FUNCTION "CAMS_PRESS" : VOID
TITLE =CAMS PRESS
AUTHOR : Esposito
FAMILY : EGAL_srl
NAME : CAMS_P
VERSION : 0.1


VAR_TEMP
  Cam_0_ON : BOOL ;
  Cam_0_OFF : BOOL ;
  Cam_1_on : BOOL ;
  Cam_1_OFF : BOOL ;
  Cam_2_ON : BOOL ;
  Cam_2_OFF : BOOL ;
  Cam_3_ON : BOOL ;
  Cam_3_OFF : BOOL ;
  Cam_4_ON : BOOL ;
  Cam_4_OFF : BOOL ;
  Cam_5_ON : BOOL ;
  Cam_5_OFF : BOOL ;
  Cam_6_ON : BOOL ;
  Cam_6_OFF : BOOL ;
  Cam_7_ON : BOOL ;
  Cam_7_OFF : BOOL ;
  Cam_8_ON : BOOL ;
  Cam_8_OFF : BOOL ;
  Cam_9_ON : BOOL ;
  Cam_9_OFF : BOOL ;
  Cam_10_ON : BOOL ;
  Cam_10_OFF : BOOL ;
  Cam_11_ON : BOOL ;
  Cam_11_OFF : BOOL ;
  Cam_12_ON : BOOL ;
  Cam_12_OFF : BOOL ;
  LD_K_parts : DINT ;
  LD_COUNT_R1 : DINT ;
  LD_COUNT_R2 : DINT ;
END_VAR
BEGIN
NETWORK
TITLE =LOAD AND TRANSFER VALUE K_PARTS COUNTERS

      U     "M_m1.0";
      SPBNB _001;
      L     "DB_TD_OP37".K_parts_counter;
      T     #LD_K_parts;
_001: NOP   0;
NETWORK
TITLE =LOAD VALUE COUNTER FROM ROBOT 1 AND 2

      U     "M_m1.0";
      =     L     16.0;
      U     L     16.0;
      SPBNB _002;
      L     "DB_SERVICE".VALUE_ROB1;
      T     #LD_COUNT_R1;
_002: NOP   0;
      U     L     16.0;
      SPBNB _003;
      L     "DB_SERVICE".VALUE_ROB2;
      T     #LD_COUNT_R2;
_003: NOP   0;
NETWORK
TITLE =COMPARE VALUES AND LOAD FORMULATION CAM_0

      U     "M_m1.0";
      =     L     16.0;
      U     L     16.0;
      U(    ;
      L     "DB_TD_OP37".Elec_Num_prog;
      L     0;
      ==I   ;
      )     ;
      U     "M_m21.1";
      =     L     16.1;
      U     L     16.1;
      SPBNB _004;
      L     "DB_TD_OP37".Elec_Start_prog;
      T     "DB_TD_OP37".Elec_cam_ON0;
_004: NOP   0;
      U     L     16.1;
      SPBNB _005;
      L     "DB_TD_OP37".Elec_Stop_prog;
      T     "DB_TD_OP37".Elec_cam_OFF0;
_005: NOP   0;
      U     L     16.0;
      U     "M_m21.1";
      U     ==0;
      =     L     16.1;
      U     L     16.1;
      U(    ;
      L     "DB_TD_OP37".Elec_Start_prog;
      L     "DB_TD_OP37".Elec_cam_ON0;
      ==I   ;
      )     ;
      =     #Cam_0_ON;
      U     L     16.1;
      U(    ;
      L     "DB_TD_OP37".Elec_Stop_prog;
      L     "DB_TD_OP37".Elec_cam_OFF0;
      ==I   ;
      )     ;
      =     #Cam_0_OFF;
      U     L     16.0;
      U     #Cam_0_ON;
      U     #Cam_0_OFF;
      R     "M_m21.1";
NETWORK
TITLE =COMPARE VALUES AND LOAD FORMULATION CAM_1

      U     "M_m1.0";
      =     L     16.0;
      U     L     16.0;
      U(    ;
      L     "DB_TD_OP37".Elec_Num_prog;
      L     1;
      ==I   ;
      )     ;
      U     "M_m21.1";
      =     L     16.1;
      U     L     16.1;
      SPBNB _006;
      L     "DB_TD_OP37".Elec_Start_prog;
      T     "DB_TD_OP37".Elec_cam_ON1;
_006: NOP   0;
      U     L     16.1;
      SPBNB _007;
      L     "DB_TD_OP37".Elec_Stop_prog;
      T     "DB_TD_OP37".Elec_cam_OFF1;
_007: NOP   0;
      U     L     16.0;
      U     "M_m21.1";
      U     ==0;
      =     L     16.1;
      U     L     16.1;
      U(    ;
      L     "DB_TD_OP37".Elec_Start_prog;
      L     "DB_TD_OP37".Elec_cam_ON1;
      ==I   ;
      )     ;
      =     #Cam_1_on;
      U     L     16.1;
      U(    ;
      L     "DB_TD_OP37".Elec_Stop_prog;
      L     "DB_TD_OP37".Elec_cam_OFF1;
      ==I   ;
      )     ;
      =     #Cam_1_OFF;
      U     L     16.0;
      U     #Cam_1_on;
      U     #Cam_1_OFF;
      R     "M_m21.1";
NETWORK
TITLE =COMPARE VALUES AND LOAD FORMULATION CAM_2

      U     "M_m1.0";
      =     L     16.0;
      U     L     16.0;
      U(    ;
      L     "DB_TD_OP37".Elec_Num_prog;
      L     2;
      ==I   ;
      )     ;
      U     "M_m21.1";
      =     L     16.1;
      U     L     16.1;
      SPBNB _008;
      L     "DB_TD_OP37".Elec_Start_prog;
      T     "DB_TD_OP37".Elec_cam_ON2;
_008: NOP   0;
      U     L     16.1;
      SPBNB _009;
      L     "DB_TD_OP37".Elec_Stop_prog;
      T     "DB_TD_OP37".Elec_cam_OFF2;
_009: NOP   0;
      U     L     16.0;
      U     "M_m21.1";
      U     ==0;
      =     L     16.1;
      U     L     16.1;
      U(    ;
      L     "DB_TD_OP37".Elec_Start_prog;
      L     "DB_TD_OP37".Elec_cam_ON2;
      ==I   ;
      )     ;
      =     #Cam_2_ON;
      U     L     16.1;
      U(    ;
      L     "DB_TD_OP37".Elec_Stop_prog;
      L     "DB_TD_OP37".Elec_cam_OFF2;
      ==I   ;
      )     ;
      =     #Cam_2_OFF;
      U     L     16.0;
      U     #Cam_2_ON;
      U     #Cam_2_OFF;
      R     "M_m21.1";
NETWORK
TITLE =COMPARE VALUES AND LOAD FORMULATION CAM_3

      U     "M_m1.0";
      =     L     16.0;
      U     L     16.0;
      U(    ;
      L     "DB_TD_OP37".Elec_Num_prog;
      L     3;
      ==I   ;
      )     ;
      U     "M_m21.1";
      =     L     16.1;
      U     L     16.1;
      SPBNB _00a;
      L     "DB_TD_OP37".Elec_Start_prog;
      T     "DB_TD_OP37".Elec_cam_ON3;
_00a: NOP   0;
      U     L     16.1;
      SPBNB _00b;
      L     "DB_TD_OP37".Elec_Stop_prog;
      T     "DB_TD_OP37".Elec_cam_OFF3;
_00b: NOP   0;
      U     L     16.0;
      U     "M_m21.1";
      U     ==0;
      =     L     16.1;
      U     L     16.1;
      U(    ;
      L     "DB_TD_OP37".Elec_Start_prog;
      L     "DB_TD_OP37".Elec_cam_ON3;
      ==I   ;
      )     ;
      =     #Cam_3_ON;
      U     L     16.1;
      U(    ;
      L     "DB_TD_OP37".Elec_Stop_prog;
      L     "DB_TD_OP37".Elec_cam_OFF3;
      ==I   ;
      )     ;
      =     #Cam_3_OFF;
      U     L     16.0;
      U     #Cam_3_ON;
      U     #Cam_3_OFF;
      R     "M_m21.1";
NETWORK
TITLE =COMPARE VALUES AND LOAD FORMULATION CAM_4

      U     "M_m1.0";
      =     L     16.0;
      U     L     16.0;
      U(    ;
      L     "DB_TD_OP37".Elec_Num_prog;
      L     4;
      ==I   ;
      )     ;
      U     "M_m21.1";
      =     L     16.1;
      U     L     16.1;
      SPBNB _00c;
      L     "DB_TD_OP37".Elec_Start_prog;
      T     "DB_TD_OP37".Elec_cam_ON4;
_00c: NOP   0;
      U     L     16.1;
      SPBNB _00d;
      L     "DB_TD_OP37".Elec_Stop_prog;
      T     "DB_TD_OP37".Elec_cam_OFF4;
_00d: NOP   0;
      U     L     16.0;
      U     "M_m21.1";
      U     ==0;
      =     L     16.1;
      U     L     16.1;
      U(    ;
      L     "DB_TD_OP37".Elec_Start_prog;
      L     "DB_TD_OP37".Elec_cam_ON4;
      ==I   ;
      )     ;
      =     #Cam_4_ON;
      U     L     16.1;
      U(    ;
      L     "DB_TD_OP37".Elec_Stop_prog;
      L     "DB_TD_OP37".Elec_cam_OFF4;
      ==I   ;
      )     ;
      =     #Cam_4_ON;
      U     L     16.0;
      U     #Cam_4_ON;
      U     #Cam_4_OFF;
      R     "M_m21.1";
NETWORK
TITLE =COMPARE VALUES AND LOAD FORMULATION CAM_5

      U     "M_m1.0";
      =     L     16.0;
      U     L     16.0;
      U(    ;
      L     "DB_TD_OP37".Elec_Num_prog;
      L     5;
      ==I   ;
      )     ;
      U     "M_m21.1";
      =     L     16.1;
      U     L     16.1;
      SPBNB _00e;
      L     "DB_TD_OP37".Elec_Start_prog;
      T     "DB_TD_OP37".Elec_cam_ON5;
_00e: NOP   0;
      U     L     16.1;
      SPBNB _00f;
      L     "DB_TD_OP37".Elec_Stop_prog;
      T     "DB_TD_OP37".Elec_cam_OFF5;
_00f: NOP   0;
      U     L     16.0;
      U     "M_m21.1";
      U     ==0;
      =     L     16.1;
      U     L     16.1;
      U(    ;
      L     "DB_TD_OP37".Elec_Start_prog;
      L     "DB_TD_OP37".Elec_cam_ON5;
      ==I   ;
      )     ;
      =     #Cam_5_ON;
      U     L     16.1;
      U(    ;
      L     "DB_TD_OP37".Elec_Stop_prog;
      L     "DB_TD_OP37".Elec_cam_OFF5;
      ==I   ;
      )     ;
      =     #Cam_5_OFF;
      U     L     16.0;
      U     #Cam_5_ON;
      U     #Cam_5_OFF;
      R     "M_m21.1";
NETWORK
TITLE =COMPARE VALUES AND LOAD FORMULATION CAM_6

      U     "M_m1.0";
      =     L     16.0;
      U     L     16.0;
      U(    ;
      L     "DB_TD_OP37".Elec_Num_prog;
      L     6;
      ==I   ;
      )     ;
      U     "M_m21.1";
      =     L     16.1;
      U     L     16.1;
      SPBNB _010;
      L     "DB_TD_OP37".Elec_Start_prog;
      T     "DB_TD_OP37".Elec_cam_ON6;
_010: NOP   0;
      U     L     16.1;
      SPBNB _011;
      L     "DB_TD_OP37".Elec_Stop_prog;
      T     "DB_TD_OP37".Elec_cam_OFF6;
_011: NOP   0;
      U     L     16.0;
      U     "M_m21.1";
      U     ==0;
      =     L     16.1;
      U     L     16.1;
      U(    ;
      L     "DB_TD_OP37".Elec_Start_prog;
      L     "DB_TD_OP37".Elec_cam_ON6;
      ==I   ;
      )     ;
      =     #Cam_6_ON;
      U     L     16.1;
      U(    ;
      L     "DB_TD_OP37".Elec_Stop_prog;
      L     "DB_TD_OP37".Elec_cam_OFF6;
      ==I   ;
      )     ;
      =     #Cam_6_OFF;
      U     L     16.0;
      U     #Cam_6_ON;
      U     #Cam_6_OFF;
      R     "M_m21.1";
NETWORK
TITLE =COMPARE VALUES AND LOAD FORMULATION CAM_7

      U     "M_m1.0";
      =     L     16.0;
      U     L     16.0;
      U(    ;
      L     "DB_TD_OP37".Elec_Num_prog;
      L     7;
      ==I   ;
      )     ;
      U     "M_m21.1";
      =     L     16.1;
      U     L     16.1;
      SPBNB _012;
      L     "DB_TD_OP37".Elec_Start_prog;
      T     "DB_TD_OP37".Elec_cam_ON7;
_012: NOP   0;
      U     L     16.1;
      SPBNB _013;
      L     "DB_TD_OP37".Elec_Stop_prog;
      T     "DB_TD_OP37".Elec_cam_OFF7;
_013: NOP   0;
      U     L     16.0;
      U     "M_m21.1";
      U     ==0;
      =     L     16.1;
      U     L     16.1;
      U(    ;
      L     "DB_TD_OP37".Elec_Start_prog;
      L     "DB_TD_OP37".Elec_cam_ON7;
      ==I   ;
      )     ;
      =     #Cam_7_ON;
      U     L     16.1;
      U(    ;
      L     "DB_TD_OP37".Elec_cam_OFF7;
      L     "DB_TD_OP37".Elec_cam_OFF2;
      ==I   ;
      )     ;
      =     #Cam_7_OFF;
      U     L     16.0;
      U     #Cam_7_ON;
      U     #Cam_7_OFF;
      R     "M_m21.1";
NETWORK
TITLE =COMPARE VALUES AND LOAD FORMULATION CAM_8

      U     "M_m1.0";
      =     L     16.0;
      U     L     16.0;
      U(    ;
      L     "DB_TD_OP37".Elec_Num_prog;
      L     8;
      ==I   ;
      )     ;
      U     "M_m21.1";
      =     L     16.1;
      U     L     16.1;
      SPBNB _014;
      L     "DB_TD_OP37".Elec_Start_prog;
      T     "DB_TD_OP37".Elec_cam_ON8;
_014: NOP   0;
      U     L     16.1;
      SPBNB _015;
      L     "DB_TD_OP37".Elec_Stop_prog;
      T     "DB_TD_OP37".Elec_cam_OFF8;
_015: NOP   0;
      U     L     16.0;
      U     "M_m21.1";
      U     ==0;
      =     L     16.1;
      U     L     16.1;
      U(    ;
      L     "DB_TD_OP37".Elec_Start_prog;
      L     "DB_TD_OP37".Elec_cam_ON8;
      ==I   ;
      )     ;
      =     #Cam_8_ON;
      U     L     16.1;
      U(    ;
      L     "DB_TD_OP37".Elec_Stop_prog;
      L     "DB_TD_OP37".Elec_cam_OFF8;
      ==I   ;
      )     ;
      =     #Cam_8_OFF;
      U     L     16.0;
      U     #Cam_8_ON;
      U     #Cam_8_OFF;
      R     "M_m21.1";
NETWORK
TITLE =COMPARE VALUES AND LOAD FORMULATION CAM_9

      U     "M_m1.0";
      =     L     16.0;
      U     L     16.0;
      U(    ;
      L     "DB_TD_OP37".Elec_Num_prog;
      L     9;
      ==I   ;
      )     ;
      U     "M_m21.1";
      =     L     16.1;
      U     L     16.1;
      SPBNB _016;
      L     "DB_TD_OP37".Elec_Start_prog;
      T     "DB_TD_OP37".Elec_cam_ON9;
_016: NOP   0;
      U     L     16.1;
      SPBNB _017;
      L     "DB_TD_OP37".Elec_Stop_prog;
      T     "DB_TD_OP37".Elec_cam_OFF9;
_017: NOP   0;
      U     L     16.0;
      U     "M_m21.1";
      U     ==0;
      =     L     16.1;
      U     L     16.1;
      U(    ;
      L     "DB_TD_OP37".Elec_Start_prog;
      L     "DB_TD_OP37".Elec_cam_ON9;
      ==I   ;
      )     ;
      =     #Cam_9_ON;
      U     L     16.1;
      U(    ;
      L     "DB_TD_OP37".Elec_Stop_prog;
      L     "DB_TD_OP37".Elec_cam_OFF9;
      ==I   ;
      )     ;
      =     #Cam_9_OFF;
      U     L     16.0;
      U     #Cam_9_ON;
      U     #Cam_9_OFF;
      R     "M_m21.1";
NETWORK
TITLE =COMPARE VALUES AND LOAD FORMULATION CAM_10

      U     "M_m1.0";
      =     L     16.0;
      U     L     16.0;
      U(    ;
      L     "DB_TD_OP37".Elec_Num_prog;
      L     10;
      ==I   ;
      )     ;
      U     "M_m21.1";
      =     L     16.1;
      U     L     16.1;
      SPBNB _018;
      L     "DB_TD_OP37".Elec_Start_prog;
      T     "DB_TD_OP37".Elec_cam_ON10;
_018: NOP   0;
      U     L     16.1;
      SPBNB _019;
      L     "DB_TD_OP37".Elec_Stop_prog;
      T     "DB_TD_OP37".Elec_cam_OFF10;
_019: NOP   0;
      U     L     16.0;
      U     "M_m21.1";
      U     ==0;
      =     L     16.1;
      U     L     16.1;
      U(    ;
      L     "DB_TD_OP37".Elec_Start_prog;
      L     "DB_TD_OP37".Elec_cam_ON10;
      ==I   ;
      )     ;
      =     #Cam_10_ON;
      U     L     16.1;
      U(    ;
      L     "DB_TD_OP37".Elec_Stop_prog;
      L     "DB_TD_OP37".Elec_cam_OFF10;
      ==I   ;
      )     ;
      =     #Cam_10_OFF;
      U     L     16.0;
      U     #Cam_10_ON;
      U     #Cam_10_OFF;
      R     "M_m21.1";
NETWORK
TITLE =COMPARE VALUES AND LOAD FORMULATION CAM_11

      U     "M_m1.0";
      =     L     16.0;
      U     L     16.0;
      U(    ;
      L     "DB_TD_OP37".Elec_Num_prog;
      L     11;
      ==I   ;
      )     ;
      U     "M_m21.1";
      =     L     16.1;
      U     L     16.1;
      SPBNB _01a;
      L     "DB_TD_OP37".Elec_Start_prog;
      T     "DB_TD_OP37".Elec_cam_ON11;
_01a: NOP   0;
      U     L     16.1;
      SPBNB _01b;
      L     "DB_TD_OP37".Elec_Stop_prog;
      T     "DB_TD_OP37".Elec_cam_OFF11;
_01b: NOP   0;
      U     L     16.0;
      U     "M_m21.1";
      U     ==0;
      =     L     16.1;
      U     L     16.1;
      U(    ;
      L     "DB_TD_OP37".Elec_Start_prog;
      L     "DB_TD_OP37".Elec_cam_ON11;
      ==I   ;
      )     ;
      =     #Cam_11_ON;
      U     L     16.1;
      U(    ;
      L     "DB_TD_OP37".Elec_Stop_prog;
      L     "DB_TD_OP37".Elec_cam_OFF11;
      ==I   ;
      )     ;
      =     #Cam_11_OFF;
      U     L     16.0;
      U     #Cam_11_ON;
      U     #Cam_11_OFF;
      R     "M_m21.1";
NETWORK
TITLE =COMPARE VALUES AND LOAD FORMULATION CAM_12

      U     "M_m1.0";
      =     L     16.0;
      U     L     16.0;
      U(    ;
      L     "DB_TD_OP37".Elec_Num_prog;
      L     12;
      ==I   ;
      )     ;
      U     "M_m21.1";
      =     L     16.1;
      U     L     16.1;
      SPBNB _01c;
      L     "DB_TD_OP37".Elec_Start_prog;
      T     "DB_TD_OP37".Elec_cam_ON12;
_01c: NOP   0;
      U     L     16.1;
      SPBNB _01d;
      L     "DB_TD_OP37".Elec_Stop_prog;
      T     "DB_TD_OP37".Elec_cam_OFF12;
_01d: NOP   0;
      U     L     16.0;
      U     "M_m21.1";
      U     ==0;
      =     L     16.1;
      U     L     16.1;
      U(    ;
      L     "DB_TD_OP37".Elec_Start_prog;
      L     "DB_TD_OP37".Elec_cam_ON12;
      ==I   ;
      )     ;
      =     #Cam_12_ON;
      U     L     16.1;
      U(    ;
      L     "DB_TD_OP37".Elec_Stop_prog;
      L     "DB_TD_OP37".Elec_cam_OFF12;
      ==I   ;
      )     ;
      =     #Cam_12_OFF;
      U     L     16.0;
      U     #Cam_12_ON;
      U     #Cam_12_OFF;
      R     "M_m21.1";
NETWORK
TITLE =ELECTRICAL CAM_0 FOR START FEEDER
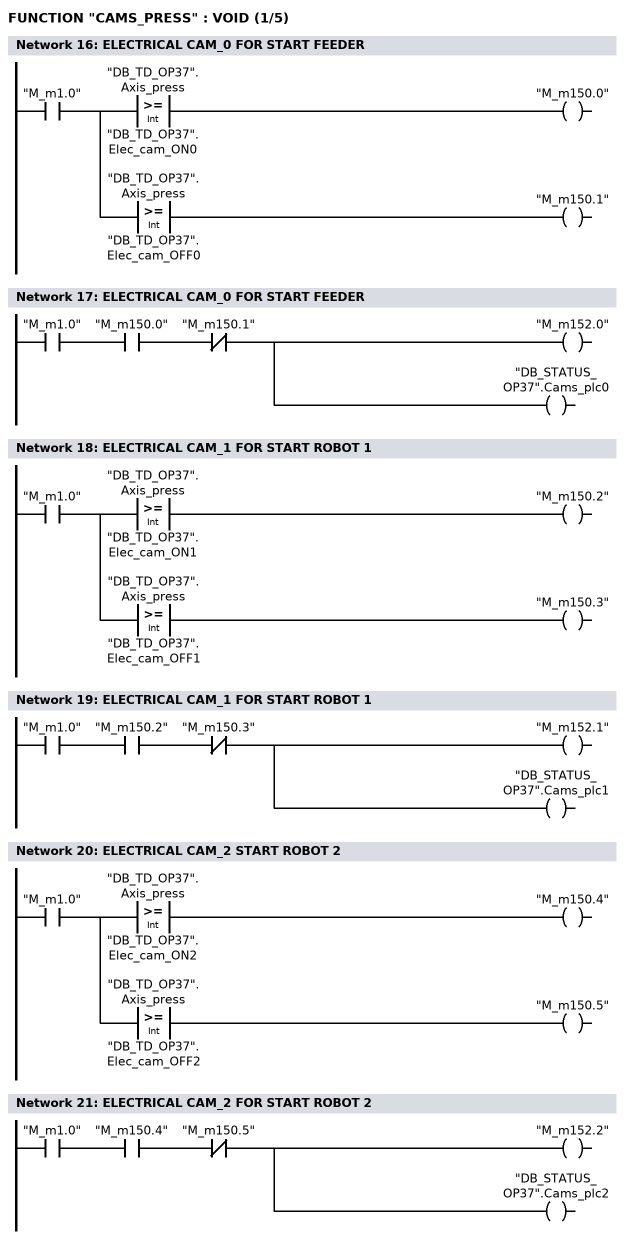
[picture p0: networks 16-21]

      U     "M_m1.0";
      =     L     16.0;
      U     L     16.0;
      U(    ;
      L     "DB_TD_OP37".Axis_press;
      L     "DB_TD_OP37".Elec_cam_ON0;
      >=I   ;
      )     ;
      =     "M_m150.0";
      U     L     16.0;
      U(    ;
      L     "DB_TD_OP37".Axis_press;
      L     "DB_TD_OP37".Elec_cam_OFF0;
      >=I   ;
      )     ;
      =     "M_m150.1";
NETWORK
TITLE =ELECTRICAL CAM_0 FOR START FEEDER

      U     "M_m1.0";
      U     "M_m150.0";
      UN    "M_m150.1";
      =     "M_m152.0";
      =     "DB_STATUS_OP37".Cams_plc0;
NETWORK
TITLE =ELECTRICAL CAM_1 FOR START ROBOT 1

      U     "M_m1.0";
      =     L     16.0;
      U     L     16.0;
      U(    ;
      L     "DB_TD_OP37".Axis_press;
      L     "DB_TD_OP37".Elec_cam_ON1;
      >=I   ;
      )     ;
      =     "M_m150.2";
      U     L     16.0;
      U(    ;
      L     "DB_TD_OP37".Axis_press;
      L     "DB_TD_OP37".Elec_cam_OFF1;
      >=I   ;
      )     ;
      =     "M_m150.3";
NETWORK
TITLE =ELECTRICAL CAM_1 FOR START ROBOT 1

      U     "M_m1.0";
      U     "M_m150.2";
      UN    "M_m150.3";
      =     "M_m152.1";
      =     "DB_STATUS_OP37".Cams_plc1;
NETWORK
TITLE =ELECTRICAL CAM_2 START ROBOT 2

      U     "M_m1.0";
      =     L     16.0;
      U     L     16.0;
      U(    ;
      L     "DB_TD_OP37".Axis_press;
      L     "DB_TD_OP37".Elec_cam_ON2;
      >=I   ;
      )     ;
      =     "M_m150.4";
      U     L     16.0;
      U(    ;
      L     "DB_TD_OP37".Axis_press;
      L     "DB_TD_OP37".Elec_cam_OFF2;
      >=I   ;
      )     ;
      =     "M_m150.5";
NETWORK
TITLE =ELECTRICAL CAM_2 FOR START ROBOT 2

      U     "M_m1.0";
      U     "M_m150.4";
      UN    "M_m150.5";
      =     "M_m152.2";
      =     "DB_STATUS_OP37".Cams_plc2;
NETWORK
TITLE =ELECTRICAL CAM_3 FOR SAFETY ROBOT 1
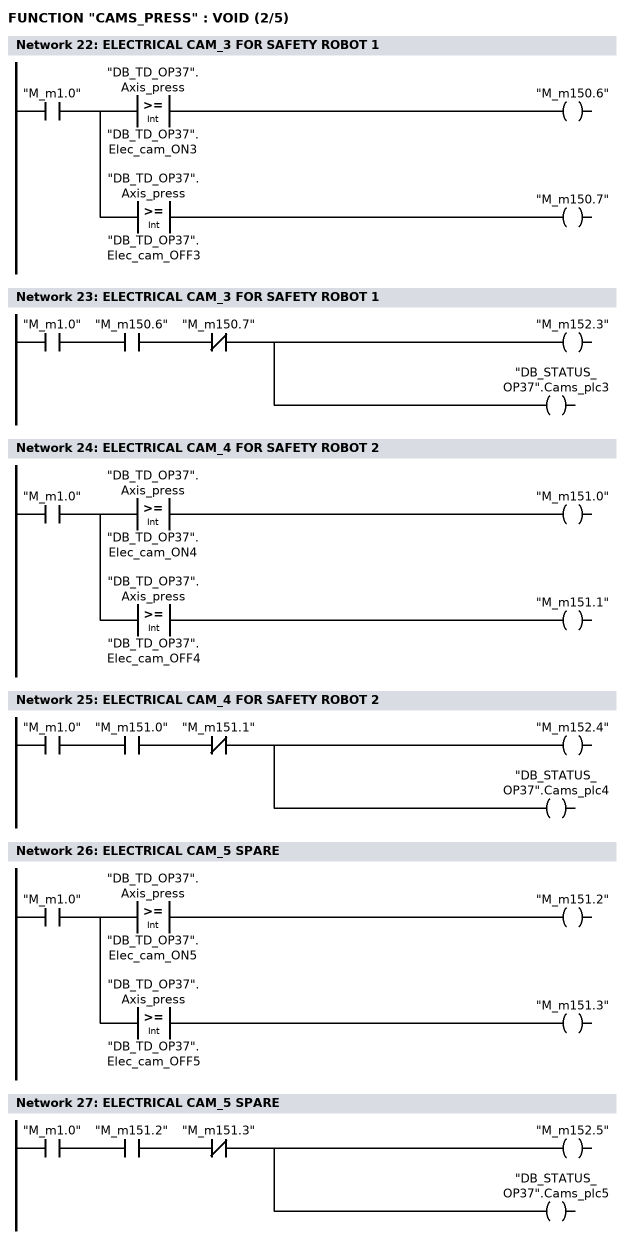
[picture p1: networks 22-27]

      U     "M_m1.0";
      =     L     16.0;
      U     L     16.0;
      U(    ;
      L     "DB_TD_OP37".Axis_press;
      L     "DB_TD_OP37".Elec_cam_ON3;
      >=I   ;
      )     ;
      =     "M_m150.6";
      U     L     16.0;
      U(    ;
      L     "DB_TD_OP37".Axis_press;
      L     "DB_TD_OP37".Elec_cam_OFF3;
      >=I   ;
      )     ;
      =     "M_m150.7";
NETWORK
TITLE =ELECTRICAL CAM_3 FOR SAFETY ROBOT 1

      U     "M_m1.0";
      U     "M_m150.6";
      UN    "M_m150.7";
      =     "M_m152.3";
      =     "DB_STATUS_OP37".Cams_plc3;
NETWORK
TITLE =ELECTRICAL CAM_4 FOR SAFETY ROBOT 2

      U     "M_m1.0";
      =     L     16.0;
      U     L     16.0;
      U(    ;
      L     "DB_TD_OP37".Axis_press;
      L     "DB_TD_OP37".Elec_cam_ON4;
      >=I   ;
      )     ;
      =     "M_m151.0";
      U     L     16.0;
      U(    ;
      L     "DB_TD_OP37".Axis_press;
      L     "DB_TD_OP37".Elec_cam_OFF4;
      >=I   ;
      )     ;
      =     "M_m151.1";
NETWORK
TITLE =ELECTRICAL CAM_4 FOR SAFETY ROBOT 2

      U     "M_m1.0";
      U     "M_m151.0";
      UN    "M_m151.1";
      =     "M_m152.4";
      =     "DB_STATUS_OP37".Cams_plc4;
NETWORK
TITLE =ELECTRICAL CAM_5 SPARE

      U     "M_m1.0";
      =     L     16.0;
      U     L     16.0;
      U(    ;
      L     "DB_TD_OP37".Axis_press;
      L     "DB_TD_OP37".Elec_cam_ON5;
      >=I   ;
      )     ;
      =     "M_m151.2";
      U     L     16.0;
      U(    ;
      L     "DB_TD_OP37".Axis_press;
      L     "DB_TD_OP37".Elec_cam_OFF5;
      >=I   ;
      )     ;
      =     "M_m151.3";
NETWORK
TITLE =ELECTRICAL CAM_5 SPARE

      U     "M_m1.0";
      U     "M_m151.2";
      UN    "M_m151.3";
      =     "M_m152.5";
      =     "DB_STATUS_OP37".Cams_plc5;
NETWORK
TITLE =ELECTRICAL CAM_6 SPARE
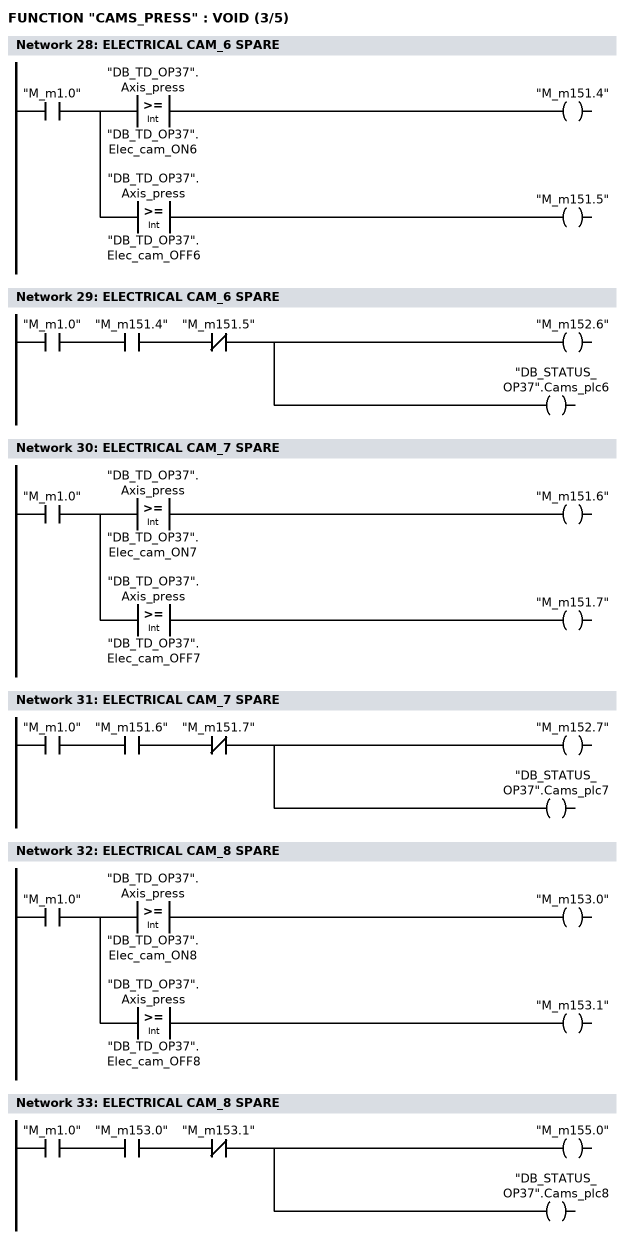
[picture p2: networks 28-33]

      U     "M_m1.0";
      =     L     16.0;
      U     L     16.0;
      U(    ;
      L     "DB_TD_OP37".Axis_press;
      L     "DB_TD_OP37".Elec_cam_ON6;
      >=I   ;
      )     ;
      =     "M_m151.4";
      U     L     16.0;
      U(    ;
      L     "DB_TD_OP37".Axis_press;
      L     "DB_TD_OP37".Elec_cam_OFF6;
      >=I   ;
      )     ;
      =     "M_m151.5";
NETWORK
TITLE =ELECTRICAL CAM_6 SPARE

      U     "M_m1.0";
      U     "M_m151.4";
      UN    "M_m151.5";
      =     "M_m152.6";
      =     "DB_STATUS_OP37".Cams_plc6;
NETWORK
TITLE =ELECTRICAL CAM_7 SPARE

      U     "M_m1.0";
      =     L     16.0;
      U     L     16.0;
      U(    ;
      L     "DB_TD_OP37".Axis_press;
      L     "DB_TD_OP37".Elec_cam_ON7;
      >=I   ;
      )     ;
      =     "M_m151.6";
      U     L     16.0;
      U(    ;
      L     "DB_TD_OP37".Axis_press;
      L     "DB_TD_OP37".Elec_cam_OFF7;
      >=I   ;
      )     ;
      =     "M_m151.7";
NETWORK
TITLE =ELECTRICAL CAM_7 SPARE

      U     "M_m1.0";
      U     "M_m151.6";
      UN    "M_m151.7";
      =     "M_m152.7";
      =     "DB_STATUS_OP37".Cams_plc7;
NETWORK
TITLE =ELECTRICAL CAM_8 SPARE

      U     "M_m1.0";
      =     L     16.0;
      U     L     16.0;
      U(    ;
      L     "DB_TD_OP37".Axis_press;
      L     "DB_TD_OP37".Elec_cam_ON8;
      >=I   ;
      )     ;
      =     "M_m153.0";
      U     L     16.0;
      U(    ;
      L     "DB_TD_OP37".Axis_press;
      L     "DB_TD_OP37".Elec_cam_OFF8;
      >=I   ;
      )     ;
      =     "M_m153.1";
NETWORK
TITLE =ELECTRICAL CAM_8 SPARE

      U     "M_m1.0";
      U     "M_m153.0";
      UN    "M_m153.1";
      =     "M_m155.0";
      =     "DB_STATUS_OP37".Cams_plc8;
NETWORK
TITLE =ELECTRICAL CAM_9 SPARE
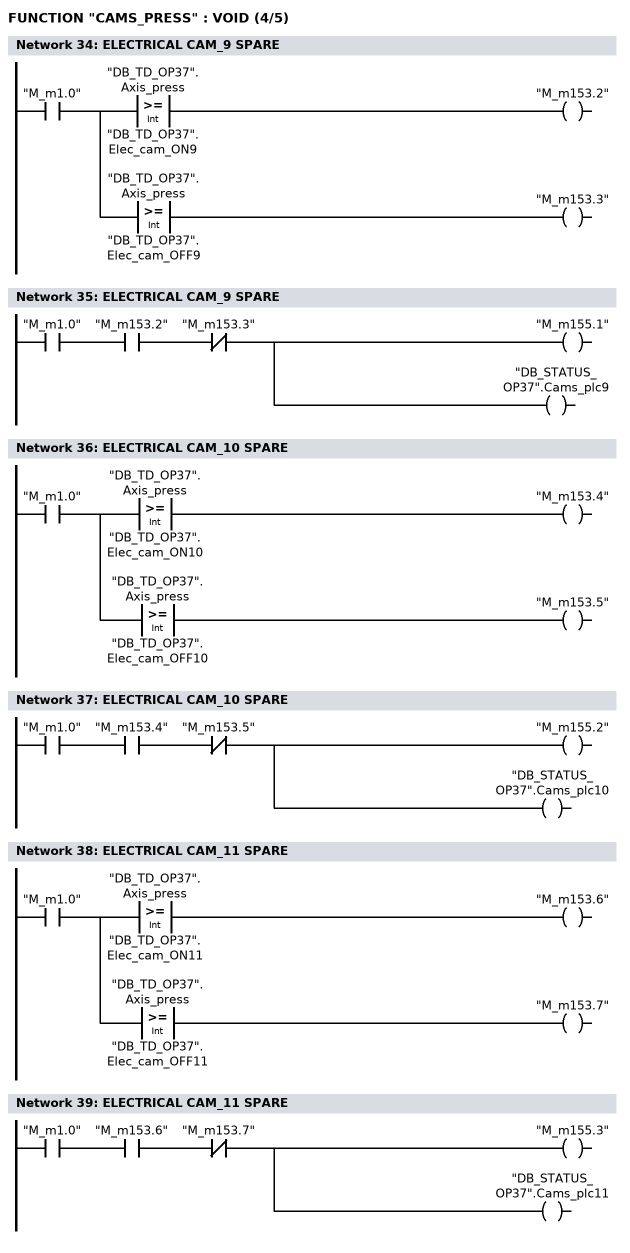
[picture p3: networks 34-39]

      U     "M_m1.0";
      =     L     16.0;
      U     L     16.0;
      U(    ;
      L     "DB_TD_OP37".Axis_press;
      L     "DB_TD_OP37".Elec_cam_ON9;
      >=I   ;
      )     ;
      =     "M_m153.2";
      U     L     16.0;
      U(    ;
      L     "DB_TD_OP37".Axis_press;
      L     "DB_TD_OP37".Elec_cam_OFF9;
      >=I   ;
      )     ;
      =     "M_m153.3";
NETWORK
TITLE =ELECTRICAL CAM_9 SPARE

      U     "M_m1.0";
      U     "M_m153.2";
      UN    "M_m153.3";
      =     "M_m155.1";
      =     "DB_STATUS_OP37".Cams_plc9;
NETWORK
TITLE =ELECTRICAL CAM_10 SPARE

      U     "M_m1.0";
      =     L     16.0;
      U     L     16.0;
      U(    ;
      L     "DB_TD_OP37".Axis_press;
      L     "DB_TD_OP37".Elec_cam_ON10;
      >=I   ;
      )     ;
      =     "M_m153.4";
      U     L     16.0;
      U(    ;
      L     "DB_TD_OP37".Axis_press;
      L     "DB_TD_OP37".Elec_cam_OFF10;
      >=I   ;
      )     ;
      =     "M_m153.5";
NETWORK
TITLE =ELECTRICAL CAM_10 SPARE

      U     "M_m1.0";
      U     "M_m153.4";
      UN    "M_m153.5";
      =     "M_m155.2";
      =     "DB_STATUS_OP37".Cams_plc10;
NETWORK
TITLE =ELECTRICAL CAM_11 SPARE

      U     "M_m1.0";
      =     L     16.0;
      U     L     16.0;
      U(    ;
      L     "DB_TD_OP37".Axis_press;
      L     "DB_TD_OP37".Elec_cam_ON11;
      >=I   ;
      )     ;
      =     "M_m153.6";
      U     L     16.0;
      U(    ;
      L     "DB_TD_OP37".Axis_press;
      L     "DB_TD_OP37".Elec_cam_OFF11;
      >=I   ;
      )     ;
      =     "M_m153.7";
NETWORK
TITLE =ELECTRICAL CAM_11 SPARE

      U     "M_m1.0";
      U     "M_m153.6";
      UN    "M_m153.7";
      =     "M_m155.3";
      =     "DB_STATUS_OP37".Cams_plc11;
NETWORK
TITLE =ELECTRICAL CAM_12 SPARE
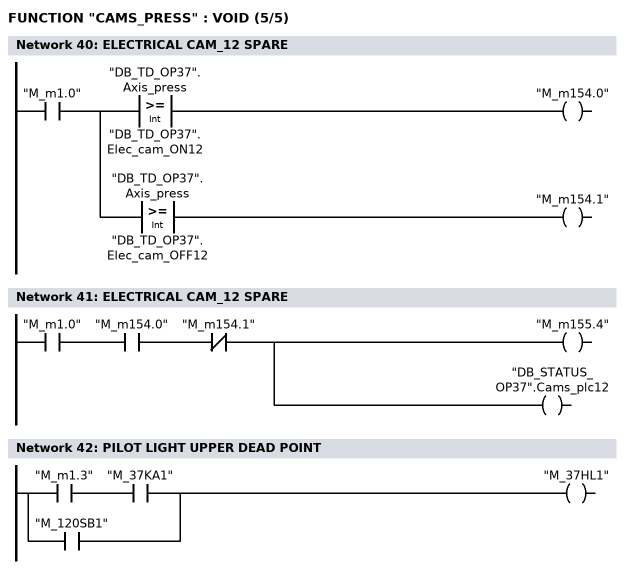
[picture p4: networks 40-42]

      U     "M_m1.0";
      =     L     16.0;
      U     L     16.0;
      U(    ;
      L     "DB_TD_OP37".Axis_press;
      L     "DB_TD_OP37".Elec_cam_ON12;
      >=I   ;
      )     ;
      =     "M_m154.0";
      U     L     16.0;
      U(    ;
      L     "DB_TD_OP37".Axis_press;
      L     "DB_TD_OP37".Elec_cam_OFF12;
      >=I   ;
      )     ;
      =     "M_m154.1";
NETWORK
TITLE =ELECTRICAL CAM_12 SPARE

      U     "M_m1.0";
      U     "M_m154.0";
      UN    "M_m154.1";
      =     "M_m155.4";
      =     "DB_STATUS_OP37".Cams_plc12;
NETWORK
TITLE =PILOT LIGHT UPPER DEAD POINT

      U     "M_m1.3";
      U     "M_37KA1";
      O     "M_120SB1";
      =     "M_37HL1";
END_FUNCTION

